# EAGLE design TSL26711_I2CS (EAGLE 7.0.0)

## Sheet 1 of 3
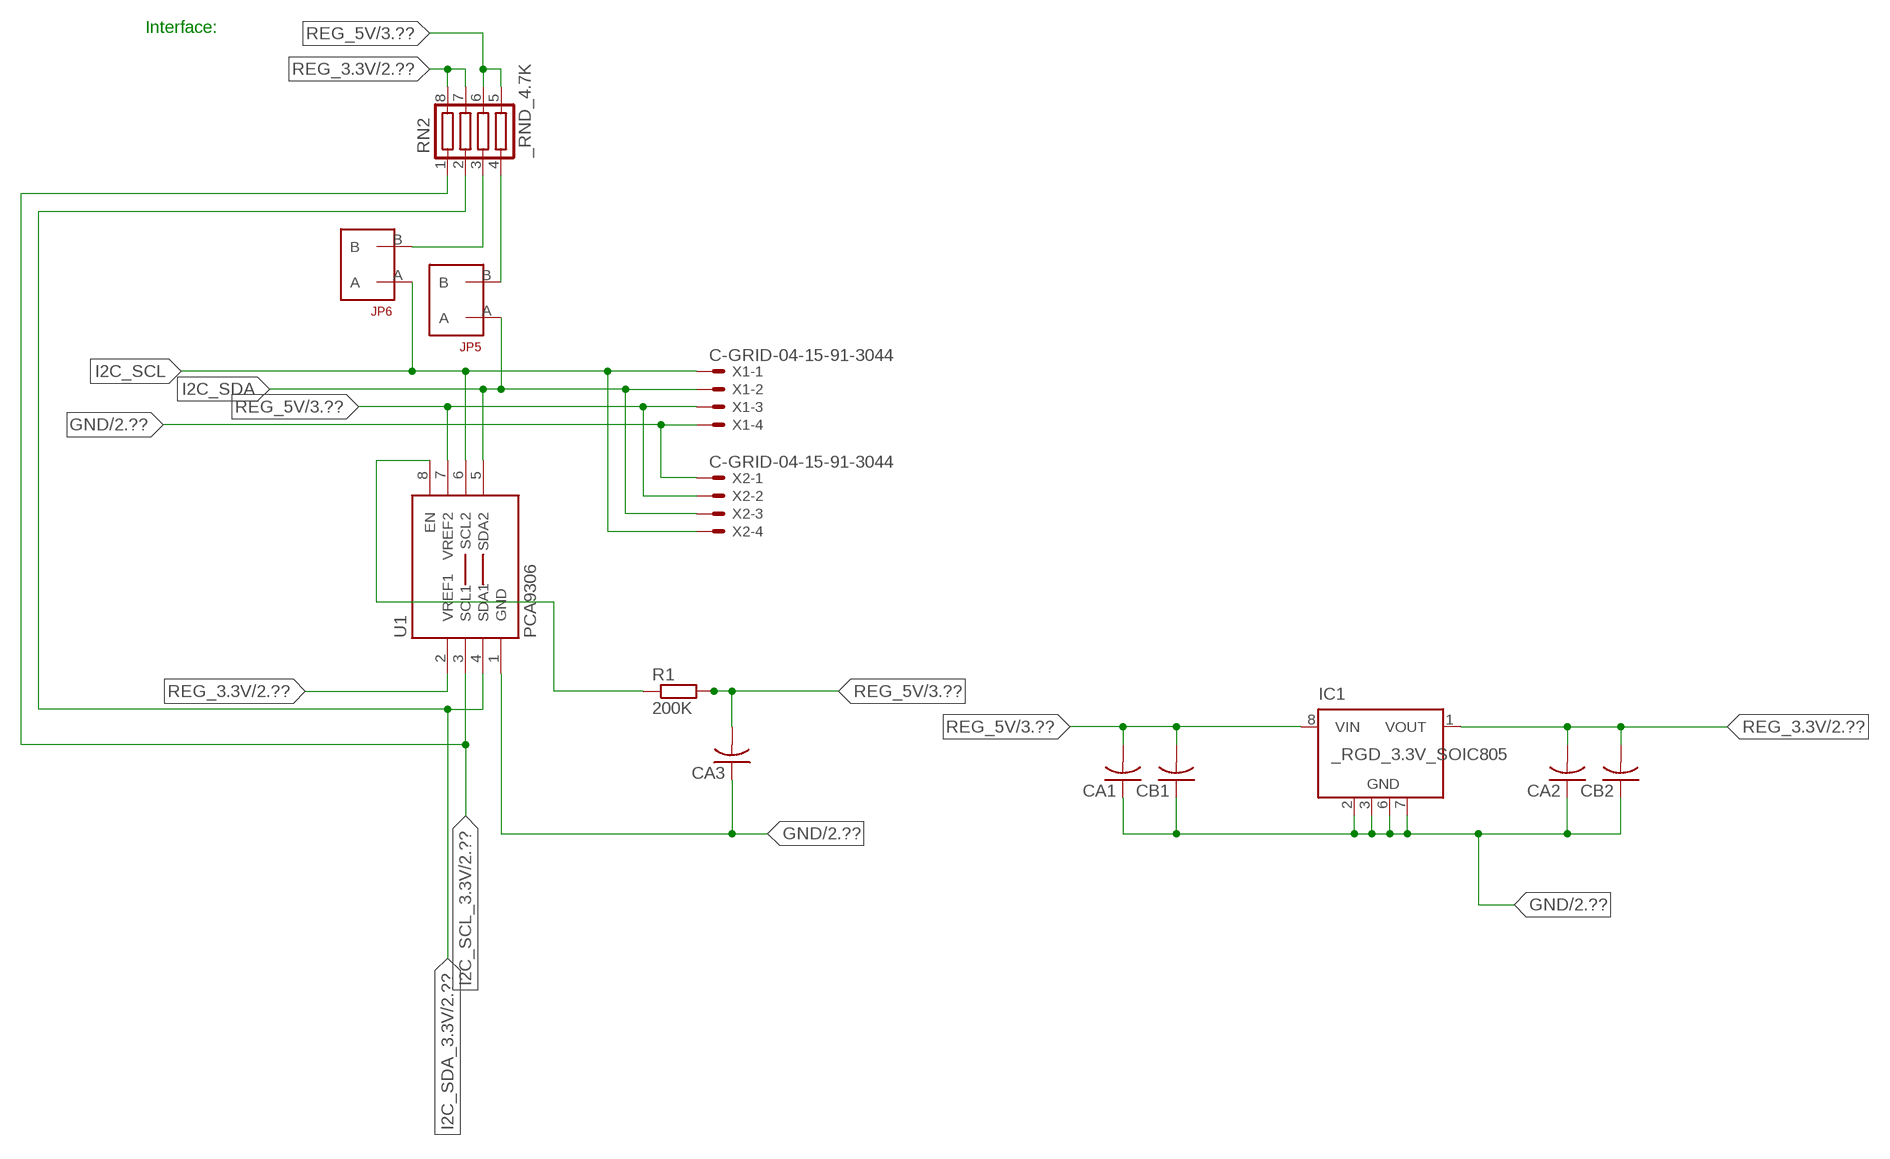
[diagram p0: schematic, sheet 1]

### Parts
CA1  CC1206KRX7R9BB104  [.1UF]
CA2  CC1206KRX7R9BB104  [.1UF]
CA3  CC1206KRX7R9BB104  [.1UF]
CB1  TMK316F106ZL-TC1206K  [TMK316F106ZL-T]
CB2  TMK316F106ZL-TC1206K  [TMK316F106ZL-T]
IC1  _RGD_3.3V_SOIC805  [_RGC_3.3V_SOIC8]
JP5  JUMPER_1X2_2MM  [JUMPER_1X2_2MM]
JP6  JUMPER_1X2_2MM  [JUMPER_1X2_2MM]
R1  200K  RESISTOR_SMT-0603  [R603]
RN2  _RND_4.7K  [RND]
U1  PCA9306  PCA9306_NCD  [PSOP-8]
X1  C-GRID-04-15-91-3044  [15-91-04]
X2  C-GRID-04-15-91-3044  [15-91-04]

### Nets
GND: CA1.1 CA2.1 CA3.1 CB1.1 CB2.1 IC1.2(GND) IC1.3(GND) IC1.6(GND) IC1.7(GND) U1.1(GND) X1.4 X2.1 ; also sheet 2,3
I2C_SCL: JP6.A U1.6(SCL2) X1.1 X2.4
I2C_SCL_3.3V: RN2.1 U1.3(SCL1) ; also sheet 2
I2C_SDA: JP5.A U1.5(SDA2) X1.2 X2.3
I2C_SDA_3.3V: RN2.2 U1.4(SDA1) ; also sheet 2
N$1: JP6.B RN2.3
N$2: JP5.B RN2.4
N$14: R1.1 U1.8(EN)
REG_3.3V: CA2.2 CB2.2 IC1.1(VOUT) RN2.7 RN2.8 U1.2(VREF1) ; also sheet 2
REG_5V: CA1.2 CA3.2 CB1.2 IC1.8(VIN) R1.2 RN2.5 RN2.6 U1.7(VREF2) X1.3 X2.2 ; also sheet 3
Unconnected: IC1.4(NC) IC1.5(NC)

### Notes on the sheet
- Interface:

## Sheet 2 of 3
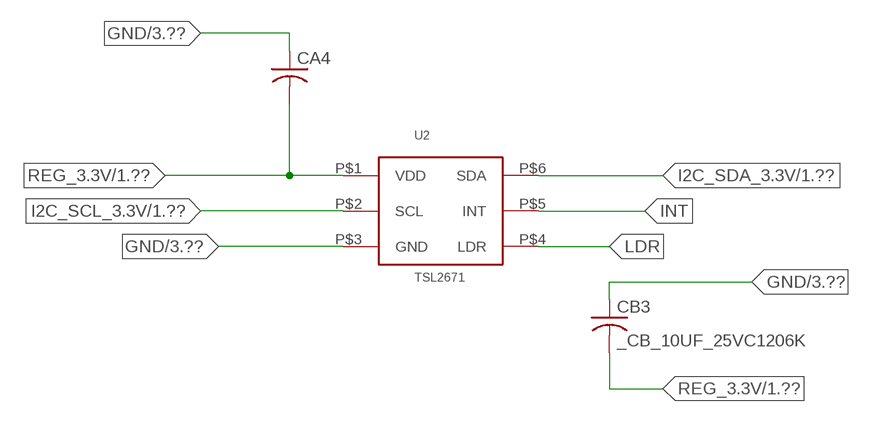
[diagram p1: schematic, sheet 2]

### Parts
CA4  _CA_.10UF_50VC1206K  [_CA_.1UF_50V]
CB3  _CB_10UF_25VC1206K  [_CB_10UF_25V]
U2  TSL2671  [TSL2771]

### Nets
GND: CA4.1 CB3.1 U2.P$3(GND) ; also sheet 1,3
I2C_SCL_3.3V: U2.P$2(SCL) ; also sheet 1
I2C_SDA_3.3V: U2.P$6(SDA) ; also sheet 1
INT: U2.P$5(INT)
LDR: U2.P$4(LDR)
REG_3.3V: CA4.2 CB3.2 U2.P$1(VDD) ; also sheet 1

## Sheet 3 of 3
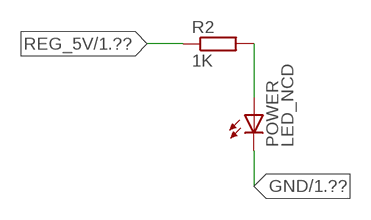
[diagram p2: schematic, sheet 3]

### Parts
POWER  LED_NCD  [CHIPLED_0603]
R2  1K  RESISTOR_SMT-0402  [R402]

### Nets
GND: POWER.C ; also sheet 1,2
N$4: POWER.A R2.2
REG_5V: R2.1 ; also sheet 1

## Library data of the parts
CA1-CA3 = NCD_ULTIMATE_LIBRARY:CC1206KRX7R9BB104: Capacitor CA .1uF 50V SMT C1206K CC1206KRX7R9BB104
CA4 = NCD_ULTIMATE_LIBRARY:_CA_.10UF_50V: Capacitor .1uF SMT
CB1 CB2 = NCD_ULTIMATE_LIBRARY:TMK316F106ZL-T: Capacitor CB 10uF SMT 1206 TMK316F106ZL-T
CB3 = NCD_ULTIMATE_LIBRARY:_CB_10UF_25V: Capacitor 10uF SMT
IC1 = NCD_ULTIMATE_LIBRARY:_RGD_3.3V_SOIC8: Regulator Linear 3.3V Chip Positive VOLTAGE REGULATOR Digikey 497-1199-2-ND/L78L33ACD13TR
JP5 JP6 = NCD_ULTIMATE_CONNECTORS:JUMPER_1X2_2MM
POWER = NCD_ULTIMATE_LIBRARY:LED_NCD: LED Digikey 754-1132-2-ND/APT2012SRCPRV
R1 R2 = NCD_ULTIMATE_LIBRARY:RESISTOR_SMT: NCD Resistor
RN2 = NCD_ULTIMATE_LIBRARY:_RND_4.7K: Resistor Array RND SMT 4.7K x 4 Single Resistor Source: http://www.ctscorp.com/components/Datasheets/CTSChipArrayDs.pdf Digikey 742C083472JPTR-ND/742C083472JP; OC_FARNELL: unknown; OC_NEWARK: unknown
U1 = NCD_ULTIMATE_LIBRARY:PCA9306_NCD: NCD Bidirectional I2C level shifter. NOT compatible with all available part number pinout schemes- DOUBLE CHECK!!!; PROD_ID: IC-10023
U2 = NCD_ULTIMATE_bhaskar:TSL2671
X1 X2 = NCD_ULTIMATE_CONNECTORS:C-GRID-04: CONNECTOR 4-Pos I2C wire to board 2.54 mm (0.100") pitch header Digikey WM1342-ND/0015912045; OC_FARNELL: unknown; OC_NEWARK: unknown

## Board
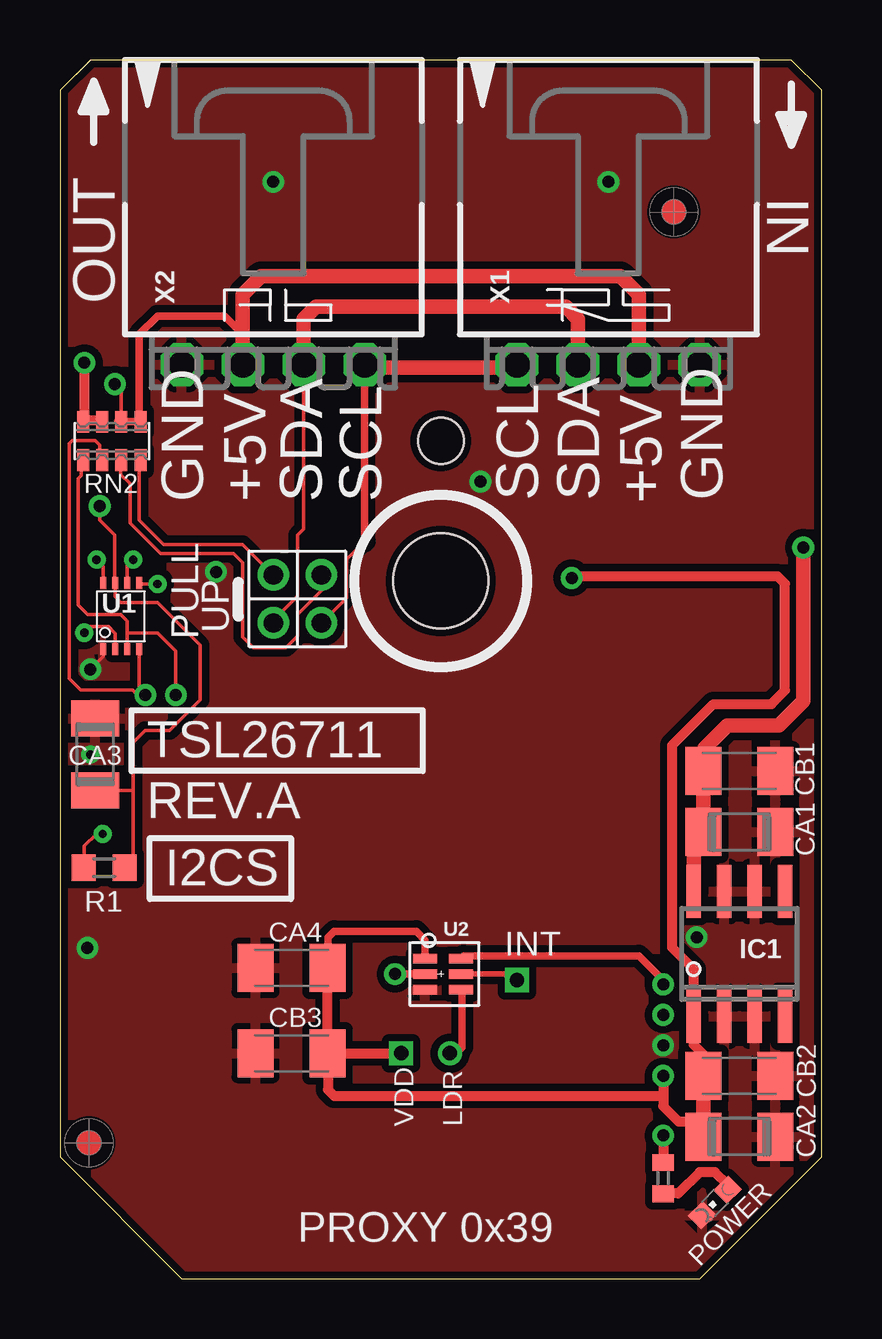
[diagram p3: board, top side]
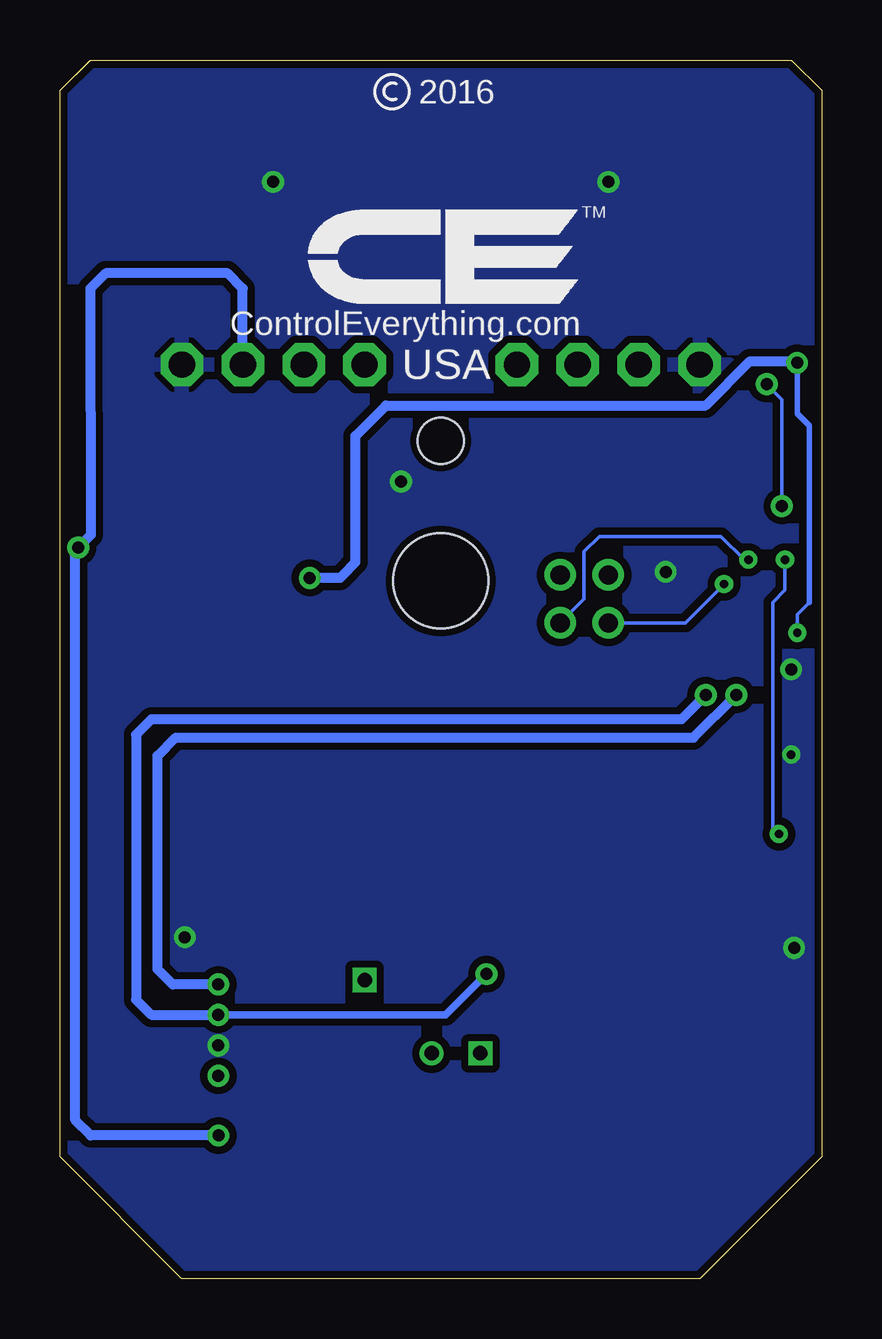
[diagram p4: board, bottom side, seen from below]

Size 31.75 x 50.8 mm. Coordinates in mm from the lower left corner, seen from the top.
Outline: 48 segments
Copper layers (1*16): Top 0.035mm / dielectric 1.5mm / Bottom 0.035mm
Design rules "default": minimum track width 5mil, minimum drill 24mil, track to track 5mil, track to pad 5mil, pad to pad 5mil, via to via 5mil, smd to smd 5mil, copper to edge 10mil, drill to drill 8mil, minimum pad ring 10mil, minimum via ring 8mil, stop-mask expansion 2mil, vias tented up to drill 0mil, thermal gap 10mil
Holes 3.96 mm at 15.88,29.08
Holes 1.91 mm at 15.88,34.93

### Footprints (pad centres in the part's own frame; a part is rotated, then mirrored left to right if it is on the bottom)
.1UF = smd 1.5 x 2: 1 -1.5,0; 2 1.5,0
_CA_.1UF_50V = smd 1.5 x 2: 1 -1.5,0; 2 1.5,0
TMK316F106ZL-T = smd 1.5 x 2: 1 -1.5,0; 2 1.5,0
_CB_10UF_25V = smd 1.5 x 2: 1 -1.5,0; 2 1.5,0
_RGC_3.3V_SOIC8 = smd 0.6 x 2.2: 1 -1.905,-2.6; 2 -0.635,-2.6; 3 0.635,-2.6; 4 1.905,-2.6; 5 1.905,2.6; 6 0.635,2.6; 7 -0.635,2.6; 8 -1.905,2.6
JUMPER_1X2_2MM = drill 0.8: A 0,2; B 0,0
CHIPLED_0603 = smd 0.8 x 0.876: A 0,-0.75; C 0,0.75
R603 = smd 1 x 1.1: 1 -0.85,0; 2 0.85,0
R402 = smd 0.7 x 0.9: 1 -0.65,0; 2 0.65,0
RND = smd 0.5 x 0.9: 1 -1.2,-0.8; 2 -0.4,-0.8; 3 0.4,-0.8; 4 1.2,-0.8; 5 1.2,0.8; 6 0.4,0.8; 7 -0.4,0.8; 8 -1.2,0.8
PSOP-8 = smd 0.25 x 0.5: 1 -0.73,-1.37; 2 -0.23,-1.37; 3 0.27,-1.37; 4 0.77,-1.37; 5 0.77,1.38; 6 0.27,1.38; 7 -0.23,1.38; 8 -0.73,1.38
TSL2771 = smd 1 x 0.4: P$1 -0.65,0.65; P$2 -0.65,0; P$3 -0.65,-0.65; P$4 0.85,-0.65; P$5 0.85,0; P$6 0.85,0.65
15-91-04 = drill 1.1 pad 1.778 octagon: 1 -3.81,-7.62; 2 -1.27,-7.62; 3 1.27,-7.62; 4 3.81,-7.62

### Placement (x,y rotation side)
CA1  28.32,18.62 180 top
CA2  28.32,5.92 180 top
CA3  1.46,21.86 270 top
CA4  9.65,12.95 0 top
CB1  28.32,21.16 180 top
CB2  28.32,8.46 180 top
CB3  9.65,9.4 0 top
IC1  28.32,13.54 0 top
JP5  8.89,29.34 180 top
JP6  10.9,29.34 180 top
POWER  27.3,3.18 135 top
R1  1.84,17.13 0 top
R2  25.15,4.19 270 top
RN2  2.16,34.93 0 top
U1  2.54,27.61 0 top
U2  15.88,12.7 0 top
U$5  [VISION_REF10]  1.21,5.66 90 top
U$28  [VISION_REF10]  25.59,44.46 90 top
X1  22.86,45.72 0 top
X2  8.89,45.72 0 top

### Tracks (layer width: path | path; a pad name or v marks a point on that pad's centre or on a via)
GND  (via drill 0.35, 0.5)
  Top 0.152: CA3.1 1.52,23.42 1.52,23.62 | v1.27,25.4 1.81,25.94 U1.1
  other vias: 8.89,45.72 22.86,45.72 25.15,9.73 17.53,33.22 26.55,14.24 1.15,13.79 6.5,29.46 1.27,21.84
  pour Top (isolate 0.305): -1.27,0 -1.27,50.8 33.02,50.8 33.02,0
  pour Bottom (isolate 0.305): -5.08,0 -5.08,50.8 35.56,50.8 35.56,0
I2C_SCL  (via drill 0.35)
  Top 0.152: 12.7,30.73 11.94,29.97 11.94,28.38 JP6.A | v3.05,29.97 2.81,29.73 U1.6
  Top 0.305: 12.7,30.73 X2.4
  Top 0.406: X2.4 12.7,37.97 | 19.05,37.97 X1.1
  Top 0.61: 12.7,37.97 19.05,37.97
  Bottom 0.152: JP6.A 9.91,28.33 9.91,30.3 9.27,30.94 4.19,30.94 3.23,29.97 v3.05,29.97
I2C_SCL_3.3V  (via drill 0.5)
  Top 0.152: RN2.1 0.89,34.07 0.89,33.48 0.77,33.35 0.77,28.08 1.16,27.69 2.54,27.69 2.81,27.42 2.81,26.92 | 2.81,26.92 U1.3 | v4.83,24.33 v4.83,24.34 4.83,26.16 4.06,26.92 2.81,26.92
  Top 0.305: U2.P$2 v13.97,12.7
  Bottom 0.305: v13.97,12.7 15.67,11 v25.15,11
  Bottom 0.406: v4.83,24.33 5.84,23.32 27.94,23.32 28.58,22.68 28.58,11.63 27.94,11 v25.15,11
I2C_SDA  (via drill 0.35)
  Top 0.152: JP5.A 8.89,27.44 9.91,28.45 9.91,30.99 10.16,31.24 10.16,34.92 X2.3 | U1.5 3.34,28.96 v4.06,28.96
  Top 0.61: X2.3 10.16,40.01 10.67,40.51 21.09,40.51 21.59,40.01 X1.2
  Bottom 0.152: v4.06,28.96 5.68,27.34 JP5.A
I2C_SDA_3.3V  (via drill 0.5)
  Top 0.152: RN2.2 1.65,34.14 1.65,34.75 1.46,34.94 0.51,34.94 0.38,34.81 0.38,26.37 0.38,26.36 0.38,25.02 0.86,24.54 3.02,24.54 3.23,24.33 v3.56,24.33 3.31,24.58 U1.4
  Top 0.305: U2.P$6 16.84,13.46 24.13,13.46 25.15,12.44 v25.15,12.27
  Bottom 0.406: v25.15,12.27 27.05,12.27 27.69,12.9 27.69,21.79 26.93,22.56 5.34,22.56 v3.56,24.33
INT  (via drill 0.6)
  Top 0.229: U2.P$5 18.54,12.7 18.8,12.45 v19.05,12.45
LDR  (via drill 0.6)
  Top 0.305: U2.P$4 16.76,11.88 16.76,9.65 16.51,9.4 v16.26,9.4
N$1
  Top 0.152: JP6.B 10.92,29.31 10.92,28.7 9.91,27.69 9.91,26.8 9.42,26.31 8.06,26.31 7.62,26.75 7.62,29.84 7.24,30.23 4.19,30.23 2.92,31.5 2.92,33.15 2.54,33.53 2.54,34.1 RN2.3
  Top 0.305: 2.54,34.02 RN2.3
N$2
  Top 0.152: JP5.B 7.62,30.61 4.32,30.61 3.3,31.62 3.3,34.07 RN2.4
  Top 0.305: 3.37,33.88 RN2.4
N$4
  Top 0.406: POWER.A 27.84,3.92 27.3,4.45 26.67,4.45 25.78,3.56 25.16,3.56 R2.2
N$14  (via drill 0.35)
  Top 0.152: R1.1 1.02,17.16 1.02,18.03 1.52,18.54 v1.78,18.54 | v1.52,29.97 1.81,29.69 U1.8
  Bottom 0.152: v1.78,18.54 2.03,18.8 2.03,28.19 1.52,28.7 v1.52,29.97
REG_3.3V  (via drill 0.35, 0.5, 0.6)
  Top 0.152: v1.02,26.92 1.27,27.18 2.03,27.18 2.31,26.9 U1.2
  Top 0.305: 11.55,13.35 11.18,13.72 11.18,14.22 11.43,14.48 14.86,14.48 15.22,14.11 U2.P$1
  Top 0.406: CB2.2 26.82,9.35 26.42,9.75 26.42,10.36 | v25.15,8.46 25.15,7.62 | 25.15,7.62 25.15,7.19 25.78,6.55 26.82,6.55 | IC1.1 26.42,12.9 25.53,13.79 25.53,22.24 27.24,23.95 29.66,23.95 30.23,24.52 30.23,28.97 29.91,29.29 21.41,29.29 v21.34,29.21 | 26.52,5.62 CA2.2 | v1.02,38.18 1.02,35.78 | 1.02,35.78 RN2.8 | 1.02,35.78 1.71,35.78 RN2.7 | 11.18,9.4 CB3.2 CA4.2 11.55,13.35 | 11.18,9.4 11.18,7.87 11.43,7.62 25.15,7.62 | 11.18,9.4 v14.22,9.4
  Top 0.61: CB2.2 26.82,6.55 CA2.2 | 26.42,10.36 IC1.1
  Bottom 0.152: 0.51,28.19 1.02,27.69 v1.02,26.92
  Bottom 0.229: 0.51,28.19 0.51,35.56 1.02,36.07 v1.02,38.18
  Bottom 0.406: v1.02,38.18 1.08,38.24 2.99,38.24 4.83,36.4 18.16,36.4 19.43,35.13 19.43,29.87 19.94,29.34 20.07,29.21 v21.34,29.21
REG_5V  (via drill 0.5)
  Top 0.152: RN2.6 2.56,37.01 v2.29,37.29 | R1.2 3.05,17.49 3.05,20.36 | 3.05,20.36 3.05,22.35 3.56,22.86 4.57,22.86 5.84,24.13 5.84,26.42 4.06,28.19 2.54,28.19 2.31,28.43 U1.7 2.29,29.01 2.29,30.99 1.65,31.62 v1.65,32.21 | CA3.2 3.05,20.36
  Top 0.305: 7.62,39.37 7.5,39.37 | 2.42,35.74 RN2.6 RN2.5 3.31,35.8 3.31,39.37 4.07,40.13 6.86,40.13 7.62,39.37 | X2.2 7.62,39.37
  Top 0.406: v25.15,5.97 R2.1
  Top 0.61: X1.3 24.13,38.23 24.13,41.02 23.37,41.78 8.38,41.78 7.62,41.02 X2.2 | IC1.8 26.42,18.21 CA1.2 CB1.2 26.86,21.2 26.86,22.11 27.82,23.06 29.98,23.06 30.99,24.08 v30.99,30.48
  Bottom 0.152: v1.65,32.21 1.65,36.65 v2.29,37.29
  Bottom 0.406: X1.3 24.13,41.28 24.77,41.91 29.84,41.91 30.48,41.27 30.47,31 v30.99,30.48 31.11,30.36 31.11,6.6 30.48,5.97 v25.15,5.97

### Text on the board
tNames: IN | OUT | GND | +5V | SDA | SCL | SCL | SDA | +5V | GND | PULL | UP | TSL26711 | REV.A | I2CS | INT | VDD | LDR | PROXY 0x39
bNames: 2016 | TM | ControlEverything.com | USA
